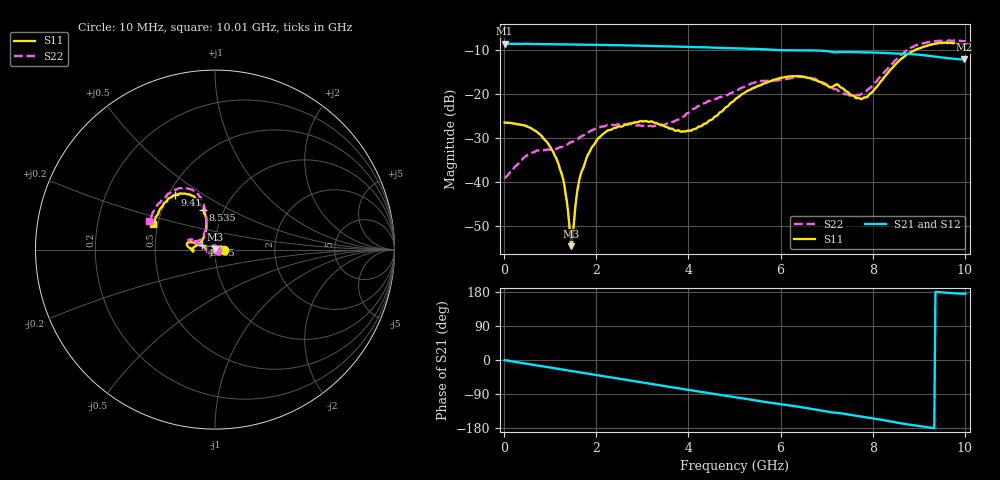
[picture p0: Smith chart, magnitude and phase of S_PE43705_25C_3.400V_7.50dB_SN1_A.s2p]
! Device ID: PE43705
! Serial: 1
! Insertion: A
! Impedance: 50 ohm
! Temp: 25C
! VDD: 3.400V
! Attenuation Step: 7.50dB
#  Hz  S  RI  R  50
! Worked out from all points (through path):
!   401 points, 10 MHz to 10.01 GHz, reference 50 ohm
!   highest |S21| = -8.53 dB at 10 MHz (marker M1); lowest = -12.1 dB at 9.985 GHz (marker M2)
!   group delay of S21, straight-line fit = 52.8 ps
!   lowest |S11| = -54.5 dB at 1.46 GHz (marker M3), VSWR 1.00, Z = 49.8 + j0.11 ohm
!   |S11| at or under -10 dB: start of sweep to 8.913 GHz
!   |S22| runs from -38.9 to -7.8 dB; largest |S21 - S12| = 0.0036
!   S11 on the Smith chart (normalised r, x): 10 MHz: 1.10, +0.00; 4.885 GHz: 0.86, +0.04; 8.535 GHz: 0.80, +0.37; 9.41 GHz: 0.54, +0.38; 10.01 GHz: 0.47, +0.16
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1e7  0.0476 4.74e-05  0.3744 -0.00181  0.3746 -0.00166  0.0113 0.000309
5.85e8  0.0374 0.0168  0.3624 -0.0767  0.3626 -0.0766  0.00522 0.021
1.01e9  0.0197 0.0149  0.3451 -0.1289  0.3452 -0.1287  -0.00873 0.0215
1.26e9  0.00834 0.00843  0.3317 -0.1571  0.3319 -0.1569  -0.0183 0.0174
1.46e9  -0.00152 0.0011  0.319 -0.1791  0.3192 -0.179  -0.0259 0.012
1.51e9  -0.00323 -0.000537  0.3155 -0.1846  0.3157 -0.1844  -0.0273 0.0109
1.61e9  -0.00814 -0.00438  0.3085 -0.1948  0.3086 -0.1947  -0.0302 0.0077
1.685e9  -0.0107 -0.00809  0.3031 -0.2025  0.3031 -0.2024  -0.0331 0.00527
1.885e9  -0.0179 -0.0159  0.2875 -0.222  0.2876 -0.2217  -0.0385 -0.00067
2.21e9  -0.0236 -0.0289  0.2592 -0.2511  0.2594 -0.251  -0.0428 -0.00893
3.36e9  -0.025 -0.0379  0.1394 -0.3211  0.1399 -0.3209  -0.0426 -0.00814
4.085e9  -0.0377 -0.0118  0.0569 -0.3377  0.0572 -0.3375  -0.0663 0.0104
4.885e9  -0.0723 0.0238  -0.0335 -0.3307  -0.0328 -0.3307  -0.0952 0.0333
5.01e9  -0.082 0.0286  -0.0472 -0.3277  -0.0468 -0.3279  -0.1024 0.0371
5.96e9  -0.145 0.0414  -0.1377 -0.2849  -0.1369 -0.2848  -0.1335 0.0544
6.685e9  -0.1475 0.0134  -0.198 -0.242  -0.1976 -0.242  -0.1412 0.0523
7.76e9  -0.0701 0.0532  -0.2567 -0.1516  -0.256 -0.1524  -0.0624 0.0798
8.36e9  -0.0501 0.1764  -0.2766 -0.0927  -0.2761 -0.094  -0.0508 0.1994
8.535e9  -0.0652 0.2197  -0.2789 -0.0734  -0.2783 -0.0764  -0.0626 0.247
9.41e9  -0.2235 0.3048  -0.264 0.00377  -0.2634 0.00333  -0.2302 0.3313
9.985e9  -0.337 0.1505  -0.2463 0.022  -0.2469 0.0218  -0.3585 0.1732
1.001e10  -0.3442 0.1418  -0.2473 0.0223  -0.2485 0.0222  -0.3662 0.1618
